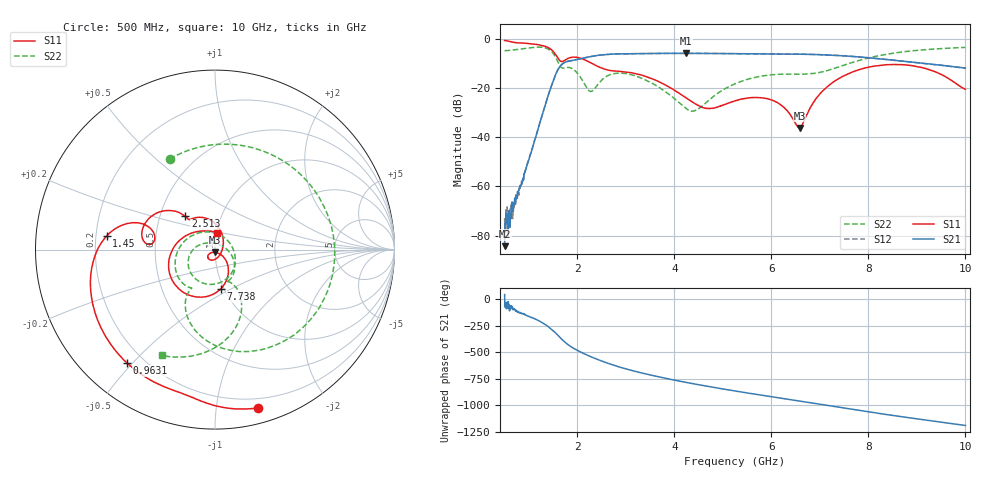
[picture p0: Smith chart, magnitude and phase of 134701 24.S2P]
!  2-Port S-parameters saved by WinCal
! VAR MeasName=S-Parameters (CALIBRATED_DATA) read from VNA (N5242A)
! VAR MeasDate=2013-7-3 16:32:02
! VAR NAME=134701 24
! VAR FILENAME=134701 24.S2P
! VAR DATE=2013-7-3 16:32:02
! VAR PHYS_PORTS=1,2
# Hz S MA R 50
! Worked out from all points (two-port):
!   1601 points, 500 MHz to 10 GHz, reference 50 ohm
!   highest |S21| = -6.00 dB at 4.235 GHz (marker M1); lowest = -84.3 dB at 500 MHz (marker M2)
!   |S21| within 3 dB of the highest: 1.864 GHz to 8.618 GHz (6.755 GHz wide, 129 % of centre)
!   lowest |S11| = -36.3 dB at 6.58 GHz (marker M3), VSWR 1.03, Z = 49.9 - j1.52 ohm
!   |S11| at or under -10 dB: 2.291 GHz to end of sweep
!   |S22| runs from -29.5 to -3.5 dB; largest |S21 - S12| = 0.0029
!   S11 on the Smith chart (normalised r, x): 500 MHz: 0.12, -1.30; 963.1 MHz: 0.14, -0.48; 1.45 GHz: 0.24, +0.06; 2.513 GHz: 0.67, +0.27; 7.738 GHz: 0.97, -0.44; 10 GHz: 1.00, +0.19
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5e8  0.914 -74.9  6.082e-05 44.6  0.0002236 -54.6  0.5646 116.6
6.840625e8  0.8354 -98.1  0.0004239 -89.9  0.0003231 -101.7  0.586 89.4
9.63125e8  0.7996 -127.9  0.002692 -155.6  0.002638 -154.5  0.6357 40.2
1.2125e9  0.7445 -156.5  0.0173 155.8  0.01756 155.6  0.6694 -15.7
1.45e9  0.6089 172.9  0.09962 83.9  0.09948 83.7  0.5648 -82.0
1.699375e9  0.3433 172.5  0.3102 -26.3  0.3097 -26.4  0.2508 -121.0
1.865625e9  0.4138 169.7  0.3552 -86.3  0.3542 -86.4  0.2525 -147.1
2.085312e9  0.3927 150.2  0.3932 -141.8  0.3923 -141.8  0.1511 149.6
2.275312e9  0.3222 137.7  0.4303 178.8  0.4297 178.8  0.08413 55.2
2.512812e9  0.2484 131.8  0.4661 135.5  0.4664 135.5  0.147 -44.3
2.94625e9  0.2122 124.9  0.4892 70.5  0.4884 70.4  0.1965 -120.7
3.670625e9  0.1341 84.4  0.4989 -11.0  0.4978 -11.0  0.1041 170.6
4.234688e9  0.06318 43.0  0.5013 -63.3  0.5008 -63.3  0.0389 108.3
4.68e9  0.03817 -18.4  0.4979 -100.6  0.4983 -100.5  0.0523 13.9
5.25e9  0.05403 -89.4  0.4922 -144.7  0.4923 -144.8  0.1203 -29.6
6.045625e9  0.05438 -137.0  0.4854 157.6  0.4849 157.6  0.1852 -62.4
6.58e9  0.01527 -93.0  0.4802 119.5  0.4807 119.4  0.189 -70.2
6.835312e9  0.04459 -40.5  0.4758 101.1  0.476 101.1  0.1934 -67.5
7.737812e9  0.2208 -81.8  0.4282 36.4  0.4289 36.2  0.3424 -64.3
8.420625e9  0.2955 -124.6  0.3711 -10.1  0.3705 -10.4  0.4888 -80.7
9.145e9  0.2514 -173.0  0.3128 -56.7  0.3118 -57.0  0.5908 -98.8
1e10  0.09327 83.2  0.2515 -110.0  0.2502 -110.2  0.6601 -116.7
